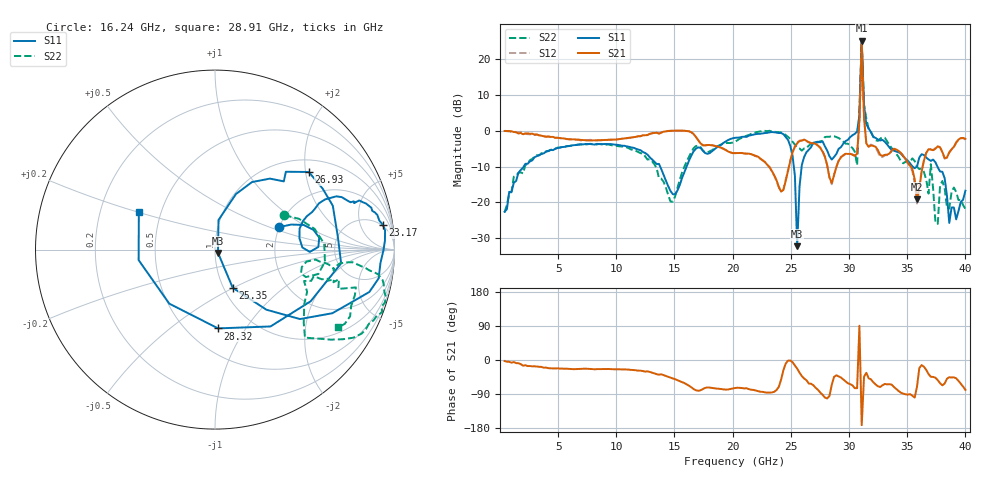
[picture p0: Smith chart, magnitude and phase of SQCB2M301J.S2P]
! Network Analyzer HP8722ES.07.66: Jul 25, 2000 Serial No. US39175408
! 27 Oct 2004  14:13:58
! Frequency  S11  S21  S12  S22
# HZ  S  DB R  50
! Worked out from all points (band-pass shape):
!   201 points, 400 MHz to 40 GHz, reference 50 ohm
!   highest |S21| = 25.01 dB at 31.09 GHz (marker M1); lowest = -19.2 dB at 35.84 GHz (marker M2)
!   |S21| within 3 dB of the highest: 31.06333 GHz to 31.11768 GHz (54.35 MHz wide, 0.175 % of centre)
!   lowest |S11| = -32.2 dB at 25.55 GHz (marker M3), VSWR 1.05, Z = 51.7 - j1.87 ohm
!   |S11| at or under -10 dB: start of sweep to 2.043 GHz; 13.76 GHz to 16.05 GHz (2.281 GHz wide, 15.3 % of centre); 37.59 GHz to end of sweep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
!   |S22| runs from -26.0 to 25.1 dB; largest |S21 - S12| = 0.69
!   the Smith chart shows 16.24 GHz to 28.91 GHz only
!   S11 on the Smith chart (normalised r, x): 16.24 GHz: 2.00, +0.59; 23.17 GHz: 5, +12; 25.35 GHz: 1.10, -0.50; 26.93 GHz: 1.30, +2.08; 28.32 GHz: 0.70, -0.76; 28.91 GHz: 0.37, +0.20
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4e8  -22.59 -100.8  -0.12 -2.8  -0.07 -2.3  -22.77 -98.7
7.132e9  -3.85 -104.3  -2.66 -22.8  -2.78 -24.1  -3.91 -121.0
1.3666e10  -9.27 -93.4  -0.86 -38.9  -0.85 -39.7  -13.23 -163.4
1.624e10  -8.41 19.3  -0.20 -67.7  -0.18 -68.6  -7.31 26.4
2.02e10  -2.00 19.7  -6.28 -74.0  -6.27 -74.1  -3.12 -6.4
2.317e10  -0.48 8.3  -10.14 -85.9  -10.27 -86.6  -0.05 -20.5
2.5348e10  -12.59 -65.1  -4.52 -14.4  -4.32 -17.5  -3.86 -39.5
2.5546e10  -32.17 -47.1  -3.53 -23.1  -3.36 -25.3  -4.70 -31.3
2.5942e10  -9.61 69.4  -2.78 -42.4  -2.71 -42.2  -5.58 -19.4
2.6932e10  -3.37 39.6  -3.55 -66.5  -3.48 -69.3  -3.70 -15.4
2.8318e10  -7.14 -87.8  -13.03 -94.9  -13.21 -94.9  -1.71 -22.5
2.8912e10  -6.51 153.9  -10.12 -40.4  -10.11 -41.8  -1.81 -32.2
3.0694e10  -0.25 43.2  -6.43 -74.3  -6.23 -75.0  -9.64 -60.8
3.0892e10  4.23 3.7  2.73 90.5  2.23 74.6  6.18 -32.7
3.109e10  24.87 -112.9  25.01 -171.8  24.82 -173.7  25.09 133.2
3.1288e10  7.17 -38.2  3.55 -44.1  3.45 -45.9  7.19 -72.2
3.1882e10  -0.47 -77.7  -4.15 -51.1  -3.90 -53.1  -0.30 -75.3
3.3466e10  -4.68 -150.7  -6.42 -63.9  -6.47 -63.0  -3.99 -126.8
3.5842e10  -10.02 -164.8  -19.16 -70.1  -20.30 -61.1  -10.06 113.5
3.802e10  -11.47 130.8  -5.97 -66.8  -6.09 -69.2  -14.03 130.4
3.8614e10  -25.71 -2.2  -6.04 -45.4  -6.14 -46.1  -21.71 137.2
4e10  -16.75 -85.9  -2.29 -78.8  -2.52 -79.2  -21.77 82.9
